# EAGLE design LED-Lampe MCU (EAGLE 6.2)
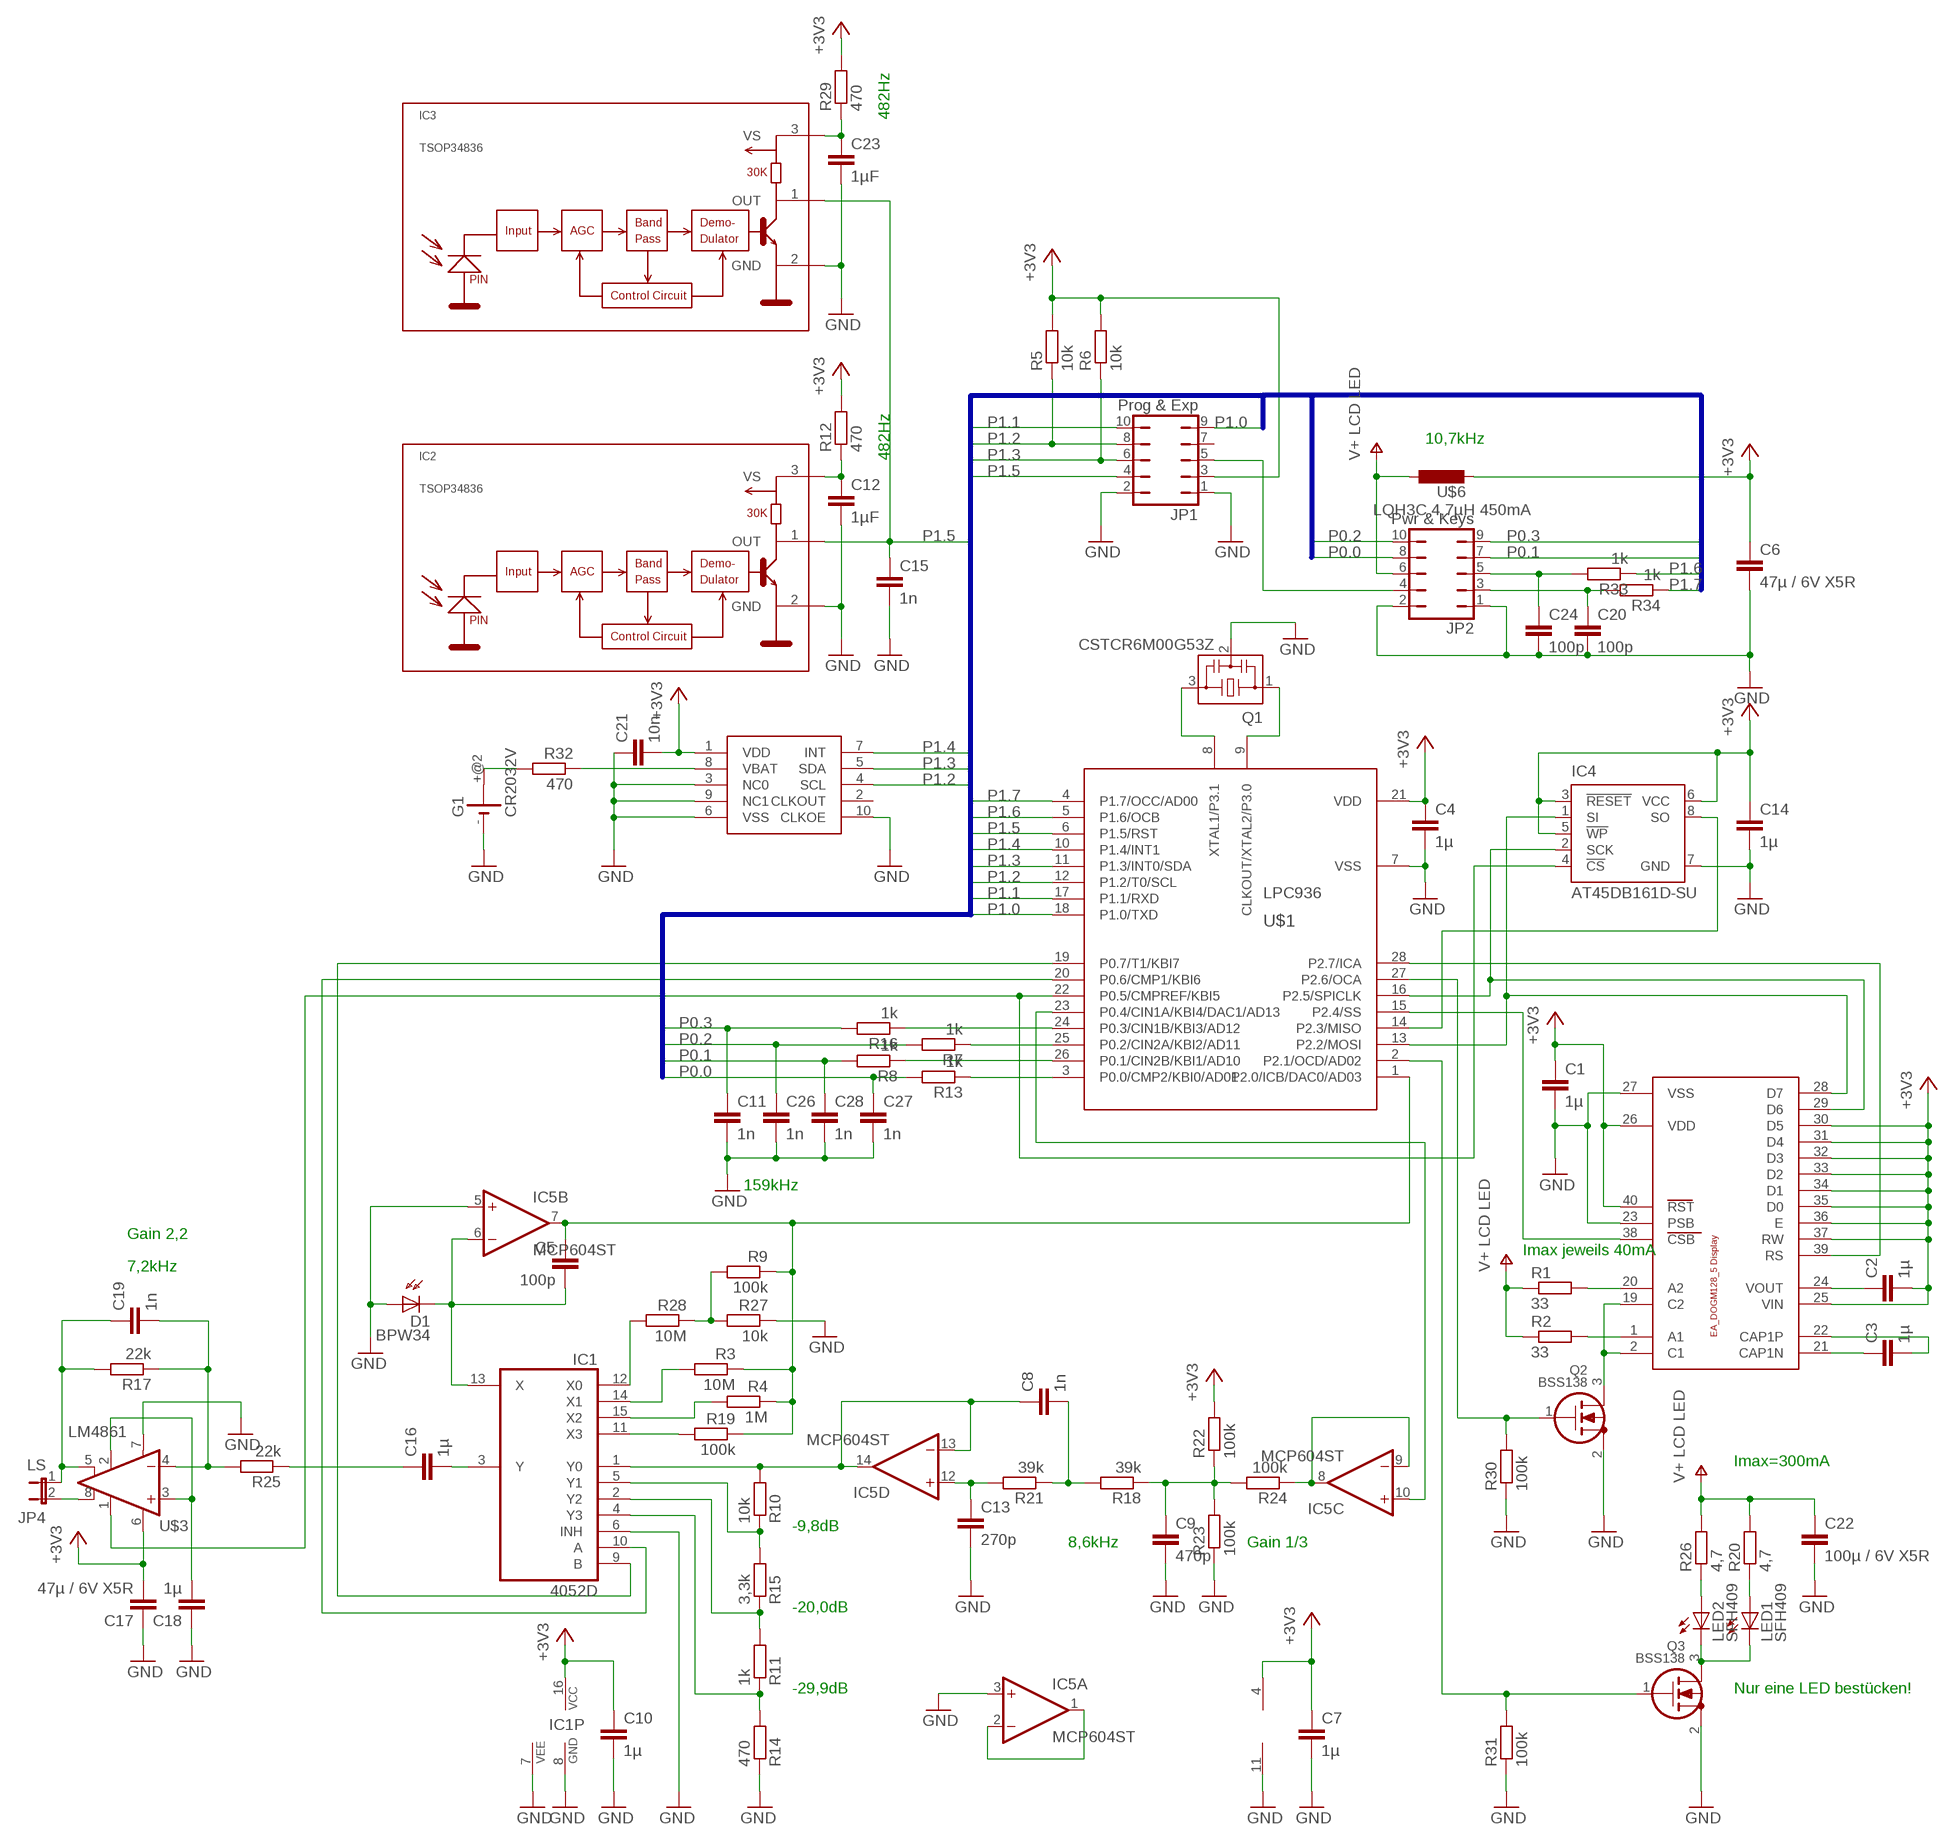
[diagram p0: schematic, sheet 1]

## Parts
C1  1µ  C-EUC0805  [C0805]
C2  1µ  C-EUC0805  [C0805]
C3  1µ  C-EUC0805  [C0805]
C4  1µ  C-EUC0805  [C0805]
C5  100p  C-EUC0603  [C0603]
C6  47µ / 6V X5R  C-EUC1206  [C1206]
C7  1µ  C-EUC0805  [C0805]
C8  1n  C-EUC0805  [C0805]
C9  470p  C-EUC0805  [C0805]
C10  1µ  C-EUC0805  [C0805]
C11  1n  C-EUC0603  [C0603]
C12  1µF  C-EUC0805  [C0805]
C13  270p  C-EUC0805  [C0805]
C14  1µ  C-EUC0805  [C0805]
C15  1n  C-EUC0603  [C0603]
C16  1µ  C-EUC1206  [C1206]
C17  47µ / 6V X5R  C-EUC1206  [C1206]
C18  1µ  C-EUC1206  [C1206]
C19  1n  C-EUC0805  [C0805]
C20  100p  C-EUC0603  [C0603]
C21  10n  C-EUC0805  [C0805]
C22  100µ / 6V X5R  C-EUC1206  [C1206]
C23  1µF  C-EUC0805  [C0805]
C24  100p  C-EUC0603  [C0603]
C26  1n  C-EUC0603  [C0603]
C27  1n  C-EUC0603  [C0603]
C28  1n  C-EUC0603  [C0603]
D1  BPW34  BPW32  [BPW32]
G1  CR2032V  [CR2032V]
IC1  4052D  [SO16]
IC2  TSOP34836  [TSOP348]
IC3  TSOP34836  [TSOP348]
IC4  AT45DB161D-SU  [8S2]
IC5  MCP604ST  [TSSOP14]
JP1  Prog & Exp  JP5Q  [JP5Q]
JP2  Pwr & Keys  JP5Q  [JP5Q]
JP4  LS  JP1E  [JP1]
LED1  SFH409  LED3MM  [LED3MM]
LED2  SFH409  LED3MM  [LED3MM]
Q1  CSTCR6M00G53Z  [CSTCR6M]
Q2  BSS138  [SOT23]
Q3  BSS138  [SOT23]
R1  33  R-EU_R1206  [R1206]
R2  33  R-EU_R1206  [R1206]
R3  10M  R-EU_R0805  [R0805]
R4  1M  R-EU_R0805  [R0805]
R5  10k  R-EU_R0805  [R0805]
R6  10k  R-EU_R0805  [R0805]
R7  1k  R-EU_R0805  [R0805]
R8  1k  R-EU_R0805  [R0805]
R9  100k  R-EU_R0805  [R0805]
R10  10k  R-EU_R0805  [R0805]
R11  1k  R-EU_R0805  [R0805]
R12  470  R-EU_R0805  [R0805]
R13  1k  R-EU_R0805  [R0805]
R14  470  R-EU_R0805  [R0805]
R15  3,3k  R-EU_R0805  [R0805]
R16  1k  R-EU_R0805  [R0805]
R17  22k  R-EU_R0805  [R0805]
R18  39k  R-EU_R0805  [R0805]
R19  100k  R-EU_R0805  [R0805]
R20  4,7  R-EU_R1206  [R1206]
R21  39k  R-EU_R0805  [R0805]
R22  100k  R-EU_R0805  [R0805]
R23  100k  R-EU_R0805  [R0805]
R24  100k  R-EU_R0805  [R0805]
R25  22k  R-EU_R0805  [R0805]
R26  4,7  R-EU_R1206  [R1206]
R27  10k  R-EU_R0805  [R0805]
R28  10M  R-EU_R0805  [R0805]
R29  470  R-EU_R0805  [R0805]
R30  100k  R-EU_R0805  [R0805]
R31  100k  R-EU_R0805  [R0805]
R32  470  R-EU_R0805  [R0805]
R33  1k  R-EU_R0805  [R0805]
R34  1k  R-EU_R0805  [R0805]
U$1  LPC936  [TSSOP28]
U$2  EA_DOGM162  [E_DOG-M162]
U$3  LM4861  [SO08]
U$4  RV3029-C2  [MC_RTC]
U$6  LQH3C 4,7µH 450mA  LQH3C  [L1210]

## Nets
+3V3: C1.1 C2.2 C4.1 C6.1 C7.1 C10.1 C14.1 C17.2 C21.2 IC1.16(VCC) IC4.3(!RESET) IC4.5(!WP) IC4.6(VCC) IC5.4(P:V+) JP1.3 R5.2 R6.2 R12.2 R22.2 R29.2 U$1.21(VDD) U$2.25(VIN) U$2.26(VDD) U$2.30(D5) U$2.31(D4) U$2.32(D3) U$2.33(D2) U$2.34(D1) U$2.35(D0) U$2.36(E) U$2.37(RW) U$2.40(RST) U$3.6(VDD) U$4.1(VDD) U$6.2
GND: C1.2 C4.2 C6.2 C7.2 C9.2 C10.2 C11.2 C12.2 C13.2 C14.2 C15.2 C17.1 C18.1 C20.2 C21.1 C22.2 C23.2 C24.2 C26.2 C27.2 C28.2 D1.A G1.- IC1.6(INH) IC1.7(VEE) IC1.8(GND) IC2.2(GND) IC3.2(GND) IC4.7(GND) IC5.3(A:+IN) IC5.5(B:+IN) IC5.11(P:V-) JP1.1 JP1.2 JP2.1 JP2.2 Q1.2 Q2.2(S) Q3.2(S) R14.1 R23.1 R27.1 R30.1 R31.1 U$1.7(VSS) U$2.23(PSB) U$2.27(VSS) U$3.7(GND) U$4.3(NC0) U$4.6(VSS) U$4.9(NC1) U$4.10(CLKOE)
N$1: C2.1 U$2.24(VOUT)
N$2: IC1.9(B) U$1.19(P0.7/T1/KBI7)
N$3: C3.2 U$2.22(CAP1P)
N$4: C3.1 U$2.21(CAP1N)
N$5: U$1.15(P2.4/SS) U$2.38(CSB)
N$6: C12.1 IC2.3(VS) R12.1
N$7: R1.2 U$2.20(A2)
N$8: R2.2 U$2.1(A1)
N$9: IC4.2(SCK) U$1.16(P2.5/SPICLK) U$2.29(D6)
N$10: IC4.1(SI) U$1.13(P2.2/MOSI) U$2.28(D7)
N$11: Q2.1(G) R30.2 U$1.27(P2.6/OCA)
N$12: IC1.10(A) U$1.20(P0.6/CMP1/KBI6)
N$13: U$1.28(P2.7/ICA) U$2.39(RS)
N$14: Q1.3 U$1.8(XTAL1/P3.1)
N$15: Q1.1 U$1.9(CLKOUT/XTAL2/P3.0)
N$16: Q2.3(D) U$2.2(C1) U$2.19(C2)
N$17: R8.1 U$1.26(P0.1/CIN2B/KBI1/AD10)
N$18: JP4.2 U$3.8(VO2)
N$19: R16.1 U$1.24(P0.3/CIN1B/KBI3/AD12)
N$20: R13.1 U$1.3(P0.0/CMP2/KBI0/AD01)
N$21: C18.2 U$3.2(BYPASS) U$3.3(+IN)
N$22: R7.1 U$1.25(P0.2/CIN2A/KBI2/AD11)
N$23: IC4.8(SO) U$1.14(P2.3/MISO)
N$25: IC1.4(Y3) R11.1 R14.2
N$26: IC1.2(Y2) R11.2 R15.1
N$27: IC1.5(Y1) R10.1 R15.2
N$28: C8.1 IC1.1(Y0) IC5.13(D:-IN) IC5.14(D:OUT) R10.2
N$29: C13.1 IC5.12(D:+IN) R21.2
N$30: C8.2 R18.2 R21.1
N$31: LED2.A R26.1
N$32: IC5.10(C:+IN) U$1.23(P0.4/CIN1A/KBI4/DAC1/AD13)
N$33: C5.2 D1.K(C) IC1.13(X) IC5.6(B:-IN)
N$34: C5.1 IC5.7(B:OUT) R3.1 R4.1 R9.1 R19.1 U$1.1(P2.0/ICB/DAC0/AD03)
N$35: IC1.11(X3) R19.2
N$36: C9.1 R18.1 R22.1 R23.2 R24.2
N$37: Q3.1(G) R31.2 U$1.2(P2.1/OCD/AD02)
N$38: IC1.15(X2) R4.2
N$39: IC1.14(X1) R3.2
N$40: IC1.12(X0) R28.2
N$41: C19.2 R17.1 R25.2 U$3.4(-IN)
N$42: C16.1 R25.1
N$43: JP1.5 JP2.4
N$44: C16.2 IC1.3(Y)
N$45: C19.1 JP4.1 R17.2 U$3.5(VO1)
N$46: LED1.K(C) LED2.K(C) Q3.3(D)
N$47: IC4.4(!CS) U$1.22(P0.5/CMPREF/KBI5) U$3.1(SHUTDOWN)
N$48: LED1.A R20.1
N$49: R32.1 U$4.8(VBAT)
N$50: R9.2 R27.2 R28.1
N$51: IC5.8(C:OUT) IC5.9(C:-IN) R24.1
N$52: G1.+@2(+) R32.2
N$53: IC5.1(A:OUT) IC5.2(A:-IN)
N$54: C23.1 IC3.3(VS) R29.1
N$55: C24.1 JP2.5 R33.2
N$56: C20.1 JP2.3 R34.2
P0.0: C27.1 JP2.8 R13.2
P0.1: C28.1 JP2.7 R8.2
P0.2: C26.1 JP2.10 R7.2
P0.3: C11.1 JP2.9 R16.2
P1.0: JP1.9 U$1.18(P1.0/TXD)
P1.1: JP1.10 U$1.17(P1.1/RXD)
P1.2: JP1.8 R5.1 U$1.12(P1.2/T0/SCL) U$4.4(SCL)
P1.3: JP1.6 R6.1 U$1.11(P1.3/INT0/SDA) U$4.5(SDA)
P1.4: U$1.10(P1.4/INT1) U$4.7(INT)
P1.5: C15.1 IC2.1(OUT) IC3.1(OUT) JP1.4 U$1.6(P1.5/RST)
P1.6: R33.1 U$1.5(P1.6/OCB)
P1.7: R34.1 U$1.4(P1.7/OCC/AD00)
V+: C22.1 JP2.6 R1.1 R2.1 R20.2 R26.2 U$6.1 ; supply symbol labelled V+ LCD LED
Unconnected: G1.+ JP1.7 U$4.2(CLKOUT)

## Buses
P1.[0..7],P0.[0..7]

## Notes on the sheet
- 482Hz
- 10,7kHz
- 482Hz
- 159kHz
- Gain 2,2
- Imax jeweils 40mA
- 7,2kHz
- Imax=300mA
- -9,8dB
- 8,6kHz | Gain 1/3
- -20,0dB
- -29,9dB | Nur eine LED bestücken!

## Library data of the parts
C1-C5 C7-C21 C23 C24 C26-C28 = rcl:C-EU: CAPACITOR, European symbol
C6 C22 = resistor:C-EU: CAPACITOR, European symbol
D1 = opto-trans-siemens:BPW32: PHOTO DIODE; OC_FARNELL: unknown; OC_NEWARK: unknown
G1 = battery:CR2032V: LI BATTERY Varta
IC1 = 40xx:4052: Dual 4-channel ANALOG MULTIPLEXER
IC2 IC3 = vishay-1:TSOP348*: IR Receiver Modules for Remote Control Systems http://www.vishay.com/ir-receiver-modules/
IC4 = atmel:AT45DB161D: 16-megabit 2.5V or 2.7V DataFlash Source: http://www.atmel.com/dyn/resources/prod_documents/doc3500.pdf; MF: ATMEL; MPN: AT45DB161D-SU; OC_FARNELL: 1455040
IC5 = linear:MCP604: Quad Op Amp 2.7V to 6.0V Single Supply CMOS Source: http://ww1.microchip.com/downloads/en/DeviceDoc/21314g.pdf
JP1 JP2 = jumper:JP5Q: JUMPER
JP4 = jumper:JP1E: JUMPER
LED1 LED2 = led:LED: LED
Q1 = murata-filter:CSTCR: Resonator Source: murata.co.jp; MPN: CSTCR6M00G53-R0; OC_FARNELL: 1170434; OC_NEWARK: 25M8759
Q2 Q3 = transistors:BSS138: BSS138: N-channel enhancement MOSFET (ON Semiconductor) 50V Uds, 200mA Id, 225mW Ptot, 3.5&Omega; Rdson
R1 R2 R5-R8 R12 R13 R16-R18 R20-R26 R29-R31 R33 R34 = rcl:R-EU_: RESISTOR, European symbol
R3 R4 R9-R11 R14 R15 R19 R27 R28 R32 = resistor:R-EU_: RESISTOR, European symbol
U$1 = nxp:LPC936
U$2 = display_ea_dog:EA_DOGM162
U$3 = LM4861:LM4861
U$4 = MicroCrystal:RV3029-C2
U$6 = mcl:LQH3C: muRata Chip Coil

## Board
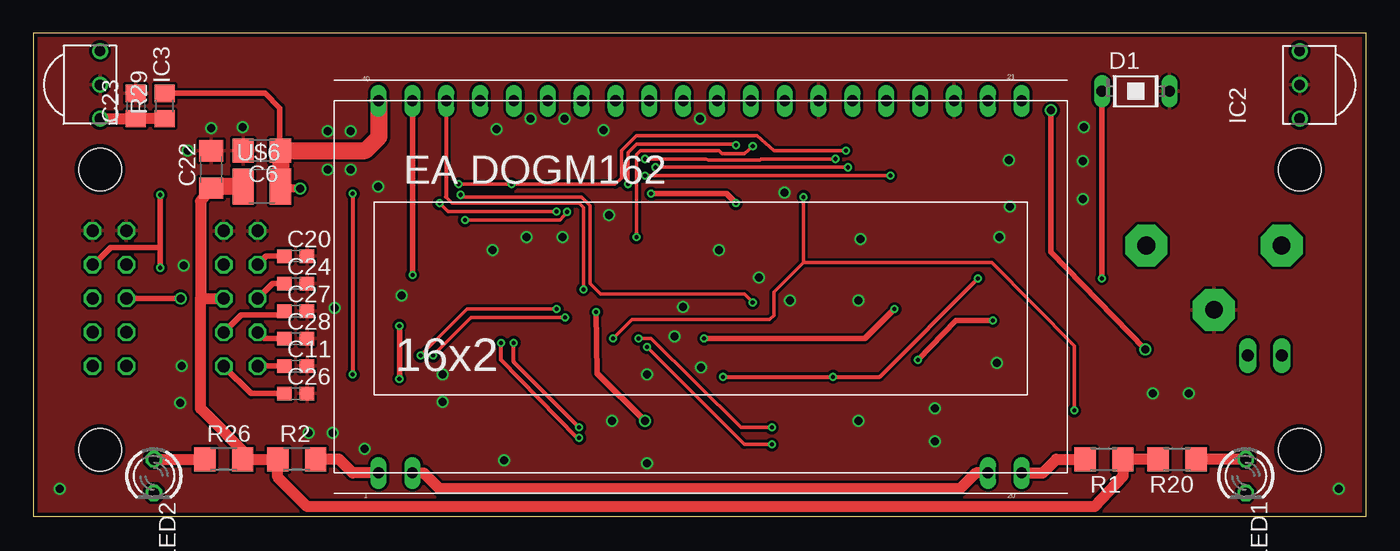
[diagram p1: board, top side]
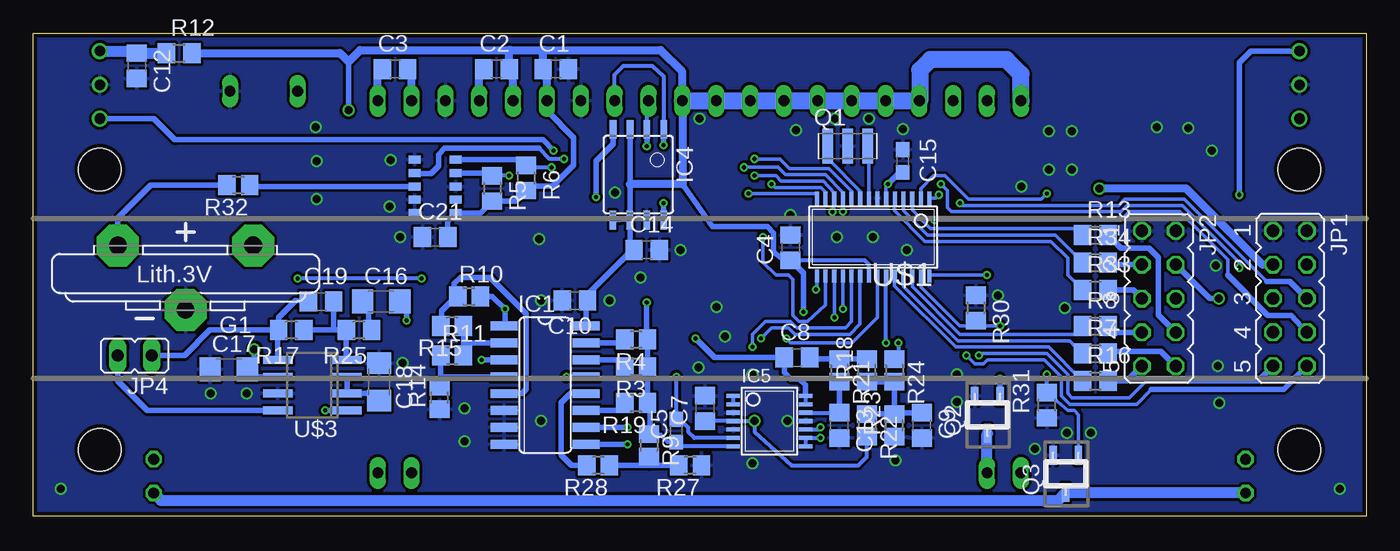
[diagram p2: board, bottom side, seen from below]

Size 100 x 36.25 mm. Coordinates in mm from the lower left corner, seen from the top.
Outline: 0,0 100,0 100,36.26 0,36.26 0,0
Copper layers (1*16): Top 0.035mm / dielectric 1.5mm / Bottom 0.035mm
Design rules: minimum track width 0.15mm, minimum drill 0.3mm, track to track 0.15mm, track to pad 0.15mm, pad to pad 0.15mm, via to via 0.15mm, smd to smd 0.15mm, copper to edge 0.3mm, drill to drill 0.2mm, minimum pad ring 0.2mm, minimum via ring 0.15mm, stop-mask expansion 0.075mm, vias tented up to drill 0mil, thermal gap 0.2mm
Holes 3.2 mm at 5,5 5,26.04 95,26.04 95,5

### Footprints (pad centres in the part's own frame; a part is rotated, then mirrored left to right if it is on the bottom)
C0805 = smd 1.3 x 1.5: 1 -0.95,0; 2 0.95,0
C0603 = smd 1.1 x 1: 1 -0.85,0; 2 0.85,0
C1206 = smd 1.6 x 1.8: 1 -1.4,0; 2 1.4,0
BPW32 = drill 0.813 long: A 0,2.54; K 0,-2.54
CR2032V = drill 1.321 pad 3.15 octagon: + -2.54,5.08; +@2 -2.54,-5.08; - 2.286,0
SO16 = smd 0.66 x 2.032: 1 -4.445,-3.073; 2 -3.175,-3.073; 3 -1.905,-3.073; 4 -0.635,-3.073; 5 0.635,-3.073; 6 1.905,-3.073; 7 3.175,-3.073; 8 4.445,-3.073; 9 4.445,3.073; 10 3.175,3.073; 11 1.905,3.073; 12 0.635,3.073; 13 -0.635,3.073; 14 -1.905,3.073; 15 -3.175,3.073; 16 -4.445,3.073
TSOP348 = drill 0.8: 1 -2.54,0; 2 0,0; 3 2.54,0
8S2 = smd 0.5 x 1.4: 1 -1.905,-3.404; 2 -0.645,-3.404; 3 0.625,-3.404; 4 1.895,-3.404; 5 1.905,3.404; 6 0.635,3.404; 7 -0.635,3.404; 8 -1.905,3.404
TSSOP14 = smd 0.305 x 0.991: 1 -1.905,-2.718; 2 -1.27,-2.718; 3 -0.635,-2.718; 4 0,-2.718; 5 0.635,-2.718; 6 1.27,-2.718; 7 1.905,-2.718; 8 1.905,2.718; 9 1.27,2.718; 10 0.635,2.718; 11 0,2.718; 12 -0.635,2.718; 13 -1.27,2.718; 14 -1.905,2.718
JP5Q = drill 0.914 octagon: 1 -5.08,-1.27; 2 -5.08,1.27; 3 -2.54,-1.27; 4 -2.54,1.27; 5 0,-1.27; 6 0,1.27; 7 2.54,-1.27; 8 2.54,1.27; 9 5.08,-1.27; 10 5.08,1.27
JP1 = drill 0.914 long: 1 0,-1.27; 2 0,1.27
LED3MM = drill 0.813 octagon: A -1.27,0; K 1.27,0
CSTCR6M = smd 0.8 x 2.6: 1 -1.5,0; 2 0,0; 3 1.5,0
SOT23 = smd 0.55 x 1.4: 1 0.95,1.4; 2 -0.95,1.4; 3 0,-1.4
R1206 = smd 1.6 x 1.803: 1 -1.422,0; 2 1.422,0
R0805 = smd 1.3 x 1.5: 1 -0.85,0; 2 0.85,0
R0805' = smd 1.3 x 1.5: 1 -0.95,0; 2 0.95,0
TSSOP28 = smd 0.305 x 0.991: 1 -4.225,-2.918; 2 -3.575,-2.918; 3 -2.925,-2.918; 4 -2.275,-2.918; 5 -1.625,-2.918; 6 -0.975,-2.918; 7 -0.325,-2.918; 8 0.325,-2.918; 9 0.975,-2.918; 10 1.625,-2.918; 11 2.275,-2.918; 12 2.925,-2.918; 13 3.575,-2.918; 14 4.225,-2.918; 15 4.225,2.918; 16 3.575,2.918; 17 2.925,2.918; 18 2.275,2.918; 19 1.625,2.918; 20 0.975,2.918; 21 0.325,2.918; 22 -0.325,2.918; 23 -0.975,2.918; 24 -1.625,2.918; 25 -2.275,2.918; 26 -2.925,2.918; 27 -3.575,2.918; 28 -4.225,2.918
E_DOG-M162 = drill 0.8 long: 1 -24.098,-13.97; 2 -21.558,-13.97; 19 21.622,-13.97; 20 24.162,-13.97; 21 24.162,13.97; 22 21.622,13.97; 23 19.082,13.97; 24 16.542,13.97; 25 14.002,13.97; 26 11.462,13.97; 27 8.922,13.97; 28 6.382,13.97; 29 3.842,13.97; 30 1.302,13.97; 31 -1.238,13.97; 32 -3.778,13.97; 33 -6.318,13.97; 34 -8.858,13.97; 35 -11.398,13.97; 36 -13.938,13.97; 37 -16.478,13.97; 38 -19.018,13.97; 39 -21.558,13.97; 40 -24.098,13.97
SO08 = smd 0.6 x 2.2: 1 -1.905,-2.6; 2 -0.635,-2.6; 3 0.635,-2.6; 4 1.905,-2.6; 5 1.905,2.6; 6 0.635,2.6; 7 -0.635,2.6; 8 -1.905,2.6
MC_RTC = smd 0.6 x 0.899: 1 -2,-1.549; 2 -1,-1.549; 3 0,-1.549; 4 1,-1.549; 5 2,-1.549; 6 2,1.549; 7 1,1.549; 8 0,1.549; 9 -1,1.549; 10 -2,1.549
L1210 = smd 1.6 x 2.7: 1 -1.4,0; 2 1.4,0

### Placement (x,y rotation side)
C1  60.8,33.58 0 bottom
C2  65.25,33.58 0 bottom
C3  72.87,33.58 0 bottom
C4  43.18,20.16 90 bottom
C5  51.75,6.43 90 bottom
C6  17.14,27.46 180 top
C7  49.61,8.1 90 bottom
C8  42.7,11.91 0 bottom
C9  33.34,6.83 270 bottom
C10  59.37,16.19 180 bottom
C11  19.68,11.27 0 top
C12  92.23,33.81 270 bottom
C13  39.53,6.83 270 bottom
C14  53.98,20 0 bottom
C15  34.77,26.67 90 bottom
C16  73.9,16.11 0 bottom
C17  85.33,11.03 0 bottom
C18  74.06,10.08 270 bottom
C19  78.42,16.11 0 bottom
C20  19.68,19.53 0 top
C21  69.85,20.95 0 bottom
C22  13.34,26.04 90 top
C23  7.7,30.8 90 top
C24  19.68,17.46 0 top
C26  19.68,9.21 0 top
C27  19.68,15.4 0 top
C28  19.68,13.34 0 top
D1  82.71,31.91 270 top
G1  88.58,17.78 270 bottom
IC1  61.59,9.84 270 bottom
IC2  95,32.38 90 top
IC3  5,32.38 270 top
IC4  54.61,25.64 180 bottom
IC5  44.77,7.14 270 bottom
JP1  5.71,16.36 270 bottom
JP2  15.56,16.35 270 bottom
JP4  92.39,12.06 90 bottom
LED1  90.96,3.02 270 top
LED2  9.05,3.02 270 top
Q1  38.89,27.78 0 bottom
Q2  28.42,7.62 0 bottom
Q3  22.54,3.17 0 bottom
R1  80.33,4.29 180 top
R2  19.76,4.29 0 top
R3  54.77,11.19 180 bottom
R4  54.77,13.26 180 bottom
R5  10k  [R0805']  65.56,24.61 270 bottom
R6  10k  [R0805']  63.02,25.4 270 bottom
R7  1k  [R0805']  20.32,12.22 0 bottom
R8  1k  [R0805']  20.32,14.29 0 bottom
R9  53.82,5.32 270 bottom
R10  67.31,16.51 0 bottom
R11  68.58,12.06 0 bottom
R12  470  [R0805']  89.06,34.77 0 bottom
R13  1k  [R0805']  20.32,21.11 0 bottom
R14  69.53,8.89 90 bottom
R15  68.58,14.29 180 bottom
R16  1k  [R0805']  20.32,10.16 0 bottom
R17  22k  [R0805']  80.64,13.97 180 bottom
R18  37.47,10.95 90 bottom
R19  54.77,8.49 180 bottom
R20  85.8,4.29 180 top
R21  39.53,10.95 270 bottom
R22  37.47,6.83 270 bottom
R23  35.4,6.83 90 bottom
R24  35.4,10.95 270 bottom
R25  22k  [R0805']  75.56,13.97 180 bottom
R26  14.29,4.29 0 top
R27  50.72,3.81 180 bottom
R28  57.63,3.81 180 bottom
R29  470  [R0805']  9.84,30.8 90 top
R30  100k  [R0805']  29.29,15.64 270 bottom
R31  100k  [R0805']  23.97,8.33 90 bottom
R32  84.61,24.84 180 bottom
R33  1k  [R0805']  20.32,16.99 0 bottom
R34  1k  [R0805']  20.32,19.05 0 bottom
U$1  36.99,20.95 180 bottom
U$2  50,17.23 0 top
U$3  79.06,9.84 90 bottom
U$4  69.85,24.77 90 bottom
U$6  17.14,24.77 0 top

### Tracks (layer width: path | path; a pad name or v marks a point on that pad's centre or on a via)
+3V3  (via drill 0.3, 0.6)
  Top 0.406: 18.57,25.21 U$6.2 | v45.88,7.14 42.31,10.72 v42.23,15.33 | v83.42,12.54 76.36,19.84 v76.36,30.48 | R29.2 17.39,31.75 18.49,30.64 18.49,27.51 C6.1
  Top 0.61: v20,24.61 19.05,24.61 18.57,25.21
  Top 1.27: U$6.2 C6.1 24.92,27.46 25.93,28.47 25.93,31.04 U$2.40
  Bottom 0.152: 51.28,31.91 51.28,32.07 U$2.30 | 55.33,22.31 IC4.6 | 33.5,31.2 U$2.37 | 42.7,18.73 C4.1 | 55.24,20.16 54.92,20.16 C14.1
  Bottom 0.305: U$1.21 37.31,18.9 37.62,19.21 C4.1 | 76.36,34.13 | R22.2 37.47,4.45 38.1,3.81 43.1,3.81 45.88,6.35 v45.88,7.14 IC5.4 49.45,7.14 C7.1
  Bottom 0.406: IC4.5 55.33,22.31 IC4.6 | C14.1 55.24,20.16 IC4.6 55.24,24.92 55.24,29.11 IC4.3 | C17.2 83.66,10.48 U$3.6 83.66,10.48 83.42,10.56 v83.42,12.54 | IC1.16 58.52,16.09 C10.1 58.42,16.67 55.24,19.84 55.24,20.16 | R5.2 66.45,22.77 U$4.1 68.9,22.17 C21.2 | C4.1 43.66,19.21 44.45,19.84 44.45,21.27 44.93,21.75 49.05,21.75 51.28,24.92 | v42.23,15.33 42.23,18.26 42.7,18.73 | v76.36,30.48 76.36,34.13 | R5.2 | R5.2 63.82,23.65 R6.2 62.71,24.77 61.04,24.77 59.45,26.35 59.45,28.42 61.44,30.4 61.44,31.17 U$2.26
  Bottom 0.61: U$2.30 51.3,33.36 52.94,35 61.67,35 | 51.28,31.91 51.28,24.92 55.24,24.92 | 64.21,35 75.49,35 76.36,34.13 76.99,34.77 R12.2 | 64.21,35 61.67,35 | v20,24.61 13.49,24.61 7.78,18.89 JP1.3 | 64.21,35 64.3,35.01 C2.2 64,33.36 U$2.25 | U$2.26 61.46,33.47 C1.1 61.75,35 61.67,35
  Bottom 1.27: U$2.30 U$2.31 U$2.32 U$2.33 U$2.34 U$2.35 U$2.36 U$2.37 | U$2.40 25.9,33.2 26.99,34.29 32.7,34.29 33.5,33.5 33.5,31.2 33.5,31.19
GND  (via drill 0.6)
  other vias: 15.72,29.21 78.82,29.21 22.07,28.89 13.34,29.13 54.45,17.94 56.75,16.19 36.99,20.95 43.18,22.62 25.88,24.77 27.62,16.59 22.07,26.04 11.59,27.46 35.32,4.21 11.11,11.27 11.03,8.49 30.72,10.64 24.84,5.08 30.72,8.57 46.04,10.64 50.09,11.19 48.74,15.72 48.1,13.49 61.91,16.19 72.47,20.95 51.44,20 86.68,9.21 83.98,9.21 61.91,7.14 72.31,11.51 23.81,26.04 1.98,2.06 73.18,26.75 73.26,23.26 39.69,20.95 34.45,20 34.77,29.05 42.78,28.97 39.85,29.84 37.31,29.84 56.36,24.29 50.01,29.84 62.07,20.8 46.04,3.97 11.27,18.81 20.64,6.27 22.46,6.27 22.62,15.64 67.63,5.64 67.63,8.1 97.95,2.06 78.74,23.81 78.74,26.67 23.81,28.89 43.42,7.14
  pour Top (isolate 0.203): 0,36.25 100,36.25 100,0 0,0
  pour Bottom (isolate 0.203): 0,0 100.01,0 100.01,36.25 0,36.25
N$1
  Bottom 0.61: U$2.24 66.54,33.07 C2.1
N$2  (via drill 0.3)
  Top 0.254: v55.4,5.4 53.34,5.4 v46.04,12.7
  Bottom 0.152: 38.6,18 U$1.19
  Bottom 0.254: v46.04,12.7 46.04,13.65 45.09,14.61 43.18,14.61 42.7,14.13 39.05,14.13 38.6,14.61 38.6,18
  Bottom 0.406: IC1.9 v55.4,5.4
N$3
  Bottom 0.61: U$2.22 71.62,33.36 C3.2
N$4
  Bottom 0.61: U$2.21 74.16,33.23 C3.1
N$5  (via drill 0.3)
  Top 0.152: U$2.38 31.01,31.33 30.96,31.27
  Top 0.254: 30.96,23.97 31.43,23.5 40.96,23.5 41.27,23.18 v41.27,17.04
  Top 0.305: 30.96,31.27 30.96,23.97
  Bottom 0.254: U$1.15 41.21,17.05 v41.27,17.04
N$6
  Bottom 0.813: IC2.3 92.32,34.92 C12.1 R12.1
N$7
  Top 0.813: U$2.20 75.73,3.26 76.76,4.29 R1.2
N$8
  Top 0.813: U$2.1 23.97,3.26 22.94,4.29 R2.2
N$9  (via drill 0.3 pad 0.3)
  Top 0.254: v53.98,27.78 53.34,27.23 51.67,27.23 51.44,27.46 45.56,27.46 45.24,27.15 v45.24,20.95
  Bottom 0.152: 53.97,27.79 v53.98,27.78 | 40.56,17.93 U$1.16
  Bottom 0.254: v45.24,20.95 45.24,19.05 44.29,18.1 43.34,18.1 43.02,17.78 43.02,15.08 42.55,14.61 41.91,14.61 40.56,15.85 40.56,17.93
  Bottom 0.305: IC4.2 53.97,31.1 U$2.29
  Bottom 0.406: IC4.2 53.97,27.79
N$10  (via drill 0.3 pad 0.3)
  Top 0.254: v44.61,24.92 44.61,27.3 45.24,27.94 52.63,27.94 v52.7,27.86
  Bottom 0.254: 52.7,29.21 IC4.1 | U$1.13 40.56,24.32 40.9,24.69 44.37,24.69 v44.61,24.92
  Bottom 0.305: U$2.28 56.38,33.15 55.72,33.81 53.58,33.81 52.7,33.02 52.7,29.21
  Bottom 0.406: v52.7,27.86 52.7,29.21
N$11  (via drill 0.3)
  Top 0.406: v27.46,10.32 v27.46,14.29
  Bottom 0.152: U$1.27 33.44,18.04
  Bottom 0.254: v27.46,14.29 29.37,14.29 30.48,14.29 33.41,17.22 33.41,18.02 33.44,18.04
  Bottom 0.305: R30.2 29.37,14.69 29.37,14.29
  Bottom 0.406: Q2.1 27.47,9.52 v27.46,10.32
N$12  (via drill 0.3)
  Top 0.254: v45.4,13.34 46.35,13.34 53.1,6.67 v55.4,6.67
  Bottom 0.152: U$1.20 37.96,18.07 37.97,18.1
  Bottom 0.254: v45.4,13.34 44.61,14.13 43.34,14.13 42.86,13.65 38.73,13.65 37.97,14.45 37.97,18.1
  Bottom 0.406: IC1.10 v55.4,6.67
N$13  (via drill 0.3)
  Top 0.406: v28.44,18.12 U$2.39
  Bottom 0.152: 32.68,18.12 U$1.28 | v28.44,18.12 28.42,18.1
  Bottom 0.254: 32.68,18.12 v28.44,18.12
N$14
  Bottom 0.152: 37.31,27.63 37.47,27.78 Q1.3
  Bottom 0.254: U$1.8 37.31,27.63
N$15
  Bottom 0.152: 40.32,26.78 40.32,27.71 Q1.1
  Bottom 0.254: U$1.9 37.96,24.42 40.32,26.78
N$16
  Top 0.813: U$2.19 70.73,3.26 69.53,2.06 30.48,2.06 29.29,3.26 U$2.2
  Bottom 0.813: U$2.2 28.44,6.2 Q2.3
N$17
  Bottom 0.152: R8.1 21.27,13.81 21.43,13.65 | 34.05,17.92 U$1.26
  Bottom 0.254: 21.43,13.65 30.48,13.65 34.05,17.25 34.05,17.92
N$18
  Bottom 0.406: JP4.2 93.66,10.16 91.44,7.94 U$3.8 81.6,7.94
N$19
  Bottom 0.152: R16.1 21.43,10.32 | U$1.24 35.36,18.06 35.38,18
  Bottom 0.254: 21.43,10.32 23.81,12.7 30.8,12.7 35.38,17.28 35.38,18
N$20
  Bottom 0.152: U$1.3 34.05,23.84
  Bottom 0.254: 34.05,23.84 34.05,22.99 32.7,21.59 21.75,21.59 R13.1
N$21
  Bottom 0.406: U$3.3 U$3.2 73.98,9.21 C18.2
N$22
  Bottom 0.152: R7.1 21.35,12.22 | 34.72,17.96 U$1.25
  Bottom 0.254: 21.35,12.22 22.23,13.18 30.64,13.18 34.72,17.25 34.72,17.96
N$23  (via drill 0.3, 0.3 pad 0.3)
  Top 0.406: v46.35,24.21 51.99,24.21 v52.7,23.5
  Bottom 0.152: U$1.14 41.21,24.07
  Bottom 0.254: 41.21,24.07 41.35,24.21 v46.35,24.21
  Bottom 0.406: v52.7,23.5 IC4.8
N$25
  Bottom 0.406: R11.1 69.43,10.32 | 69.43,10.32 69.43,9.84 R14.2 | IC1.4 69.27,10.48 69.43,10.32
N$26
  Bottom 0.406: IC1.2 67.63,13.02 67.63,12.17 R11.2 R15.1
N$27
  Bottom 0.406: IC1.5 63.34,9.21 63.02,9.53 63.02,15.24 65.72,17.94 67.94,17.94 68.42,17.46 68.42,16.57 R10.1 68.26,16.51 69.37,15.4 69.37,14.45 69.53,14.29 R15.2 69.37,14.29
N$28  (via drill 0.3)
  Top 0.406: v50.32,13.34 62.39,13.34 v64.61,15.56
  Bottom 0.305: IC5.13 IC5.14
  Bottom 0.406: R10.2 65.56,16.51 v64.61,15.56 | v64.61,15.56 64.61,14.35 IC1.1 | v50.32,13.34 48.9,11.91 C8.1 43.65,10.79 43.18,10.32 42.55,10.32 42.07,9.84 42.07,9.07 IC5.14 | v64.61,15.56 64.61,14.29
N$29
  Bottom 0.305: IC5.12 39.69,7.78 C13.1
  Bottom 0.406: 39.85,7.94 C13.1 R21.2
N$30
  Bottom 0.152: 42.07,11.91 41.91,11.91 41.75,11.8
  Bottom 0.254: 41.75,11.8 41.97,11.96
  Bottom 0.406: R18.2 R21.1 41.75,11.8 | C8.2 42.07,11.91
N$31
  Top 0.305: 12.78,4.29 R26.1
  Top 0.813: LED2.A 12.78,4.29
N$32  (via drill 0.3)
  Top 0.305: v40.96,6.67 36.04,11.59 v36.04,13.02
  Bottom 0.305: IC5.10 41.12,6.51 v40.96,6.67 | v36.04,13.02 36.04,18.1 U$1.23
N$33  (via drill 0.3)
  Top 0.305: v51.75,10.48 v60.01,10.48 63.5,10.48 v70.88,17.86
  Top 0.406: v80.17,17.86 D1.K
  Bottom 0.305: v70.88,17.86 v80.17,17.86 | v51.75,10.48 C5.2 51.49,7.28 50.88,6.67 50.88,6.35 50.4,5.87 IC5.6
  Bottom 0.406: v60.01,10.48 IC1.13
N$34  (via drill 0.3 pad 0.3)
  Top 0.254: v32.07,24.13 32.23,23.97 41.12,23.97 41.75,23.34 41.75,17.46 42.55,16.67 53.34,16.67 v53.98,16.03
  Bottom 0.152: 53.98,13.71 R4.1
  Bottom 0.254: U$1.1 32.27,23.87 v32.07,24.13
  Bottom 0.305: IC5.7 51.41,5.24 C5.1 52.41,5.58 52.94,6.11 53.76,6.11 R9.1
  Bottom 0.406: R4.1 R3.1 R19.1 53.74,8.49 53.74,6.19 R9.1 | v53.98,16.03 53.98,13.71
N$35
  Bottom 0.406: R19.2 56.12,7.94 IC1.11
N$36
  Bottom 0.406: 35.72,10.16 R24.2 | R18.1 R24.2 | R24.2 R23.2 | R23.2 R22.1 | C9.1 35.32,7.78 35.4,7.78 R23.2
N$37  (via drill 0.3)
  Top 0.305: v23.97,24.21 v23.97,10.64
  Bottom 0.254: U$1.2 33.41,24.61 32.46,25.56 31.59,25.56 29.84,23.81 24.37,23.81 v23.97,24.21 | R31.2 22.38,7.94 21.91,7.94 21.59,7.62 21.59,4.6
  Bottom 0.305: 21.59,4.6 Q3.1 | R31.2 v23.97,10.64
  Bottom 0.406: R31.2
N$38
  Bottom 0.406: IC1.15 55.8,13.02 R4.2
N$39
  Bottom 0.406: R3.2 55.88,11.59 55.88,11.75 IC1.14
N$40
  Bottom 0.406: R28.2 59.61,3.81 60.4,4.6 60.4,8.49 59.69,9.21 IC1.12
N$41
  Bottom 0.406: R17.1 R25.2 | C19.2 77.47,13.97 R25.2 | R25.2 76.52,11.8 U$3.4
N$42
  Bottom 0.406: R25.1 74.85,13.97 74.85,16.11 C16.1
N$43  (via drill 0.6)
  Top 0.406: JP1.5 v11.04,16.36
  Bottom 0.406: v11.04,16.36 11.75,16.35 JP2.4
N$44  (via drill 0.3)
  Top 0.406: v66.36,11.75 69.22,14.68 v71.99,14.68
  Bottom 0.406: IC1.3 v66.36,11.75 | v71.99,14.68 71.99,16.11 C16.2
N$45
  Bottom 0.406: U$3.5 81.66,13.91 R17.2 | R17.2 81.59,14.93 80.33,16.19 C19.1 | JP4.1 88.66,12.06 86.76,13.97 R17.2
N$46
  Bottom 0.813: LED2.K 22.51,1.75 Q3.3 22.57,1.75 23.1,1.19 90.41,1.19 LED1.K
N$47  (via drill 0.3)
  Top 0.254: v43.5,13.34 44.93,14.76 55.24,14.76 55.56,15.08 55.56,16.83 57.78,19.05 | 57.78,19.05 v57.78,23.97 | 57.78,19.05 71.91,19.05 78.11,12.78 v78.11,7.94
  Bottom 0.152: U$1.22 | IC4.4 56.51,29.06 IC4.4
  Bottom 0.254: U$1.22 36.66,14.93 38.58,13.02 43.18,13.02 v43.5,13.34
  Bottom 0.406: v57.78,23.97 57.78,26.67 56.52,27.94 IC4.4 | v78.11,7.94 U$3.1
N$48
  Top 0.813: LED1.A R20.1
N$49
  Bottom 0.406: U$4.8 83.68,24.77 R32.1
N$50
  Bottom 0.406: R27.2 53.74,3.81 | 53.74,3.81 R28.1 | R9.2 53.74,4.45 53.74,3.81
N$51  (via drill 0.3)
  Top 0.305: v40.96,5.87 40.8,5.87 35.08,11.75 v35.08,13.02
  Bottom 0.305: IC5.8 IC5.9 v40.96,5.87 | v35.08,13.02 35.08,11.8 R24.1
N$52
  Bottom 0.406: R32.2 91.2,24.84 93.66,22.38 G1.+@2
N$53
  Bottom 0.305: IC5.2 IC5.1
N$54
  Top 0.813: C23.1 | IC3.3 C23.1 | R29.1 C23.1
N$55
  Top 0.406: C24.1 17.94,17.46 JP2.5
  Bottom 0.406: JP2.5 17.46,16.98 R33.2
N$56
  Top 0.406: C20.1 17.47,19.53 JP2.3
  Bottom 0.406: JP2.3 18.9,18.89 R34.2
P0.0
  Top 0.406: 18.89,15.4 C27.1 18.78,15.4 18.49,15.11 15.59,15.11 JP2.8
  Bottom 0.406: JP2.8 15.6,15.12 15.6,19.43 16.31,20.14 18.4,20.14 R13.2
P0.1
  Top 0.152: JP2.7
  Top 0.406: C28.1 17.3,13.34 JP2.7
  Bottom 0.152: R8.2 | JP2.7 16.84,13.79
  Bottom 0.406: R8.2 18.89,13.81 JP2.7
P0.2
  Top 0.406: C26.1 16.35,9.21 JP2.10
  Bottom 0.152: 18.73,12.38 R7.2
  Bottom 0.406: JP2.10 15.4,12.38 18.73,12.38
P0.3
  Top 0.152: JP2.9
  Top 0.406: C11.1 JP2.9
  Bottom 0.406: JP2.9 17.94,10.16 R16.2
P1.0  (via drill 0.3, 0.3 pad 0.3)
  Top 0.254: v39.26,15.56 32.54,15.56 v29.05,12.06
  Bottom 0.152: 39.26,17.98 U$1.18 | v29.05,12.06 28.89,12.22
  Bottom 0.254: v39.26,15.56 39.26,17.98 | 28.89,12.22 23.97,12.22 22.38,10.64 22.38,9.21 22.07,8.89 17.78,8.89 16.51,10.16
  Bottom 0.406: 16.51,10.16 8.1,10.16 JP1.9
P1.1  (via drill 0.3, 0.3 pad 0.3)
  Top 0.254: v30,12.06 32.86,14.92 v39.9,14.92
  Bottom 0.152: 39.9,17.95 U$1.17 | JP1.10
  Bottom 0.254: v39.9,14.92 39.9,17.95 | 16.11,9.53 17.22,8.41 22.23,8.41 22.86,9.05 22.86,10.48 24.13,11.75 28.42,11.75 28.73,11.43 29.37,11.43 v30,12.06
  Bottom 0.406: JP1.10 6.19,9.53 16.11,9.53
P1.2  (via drill 0.3)
  Top 0.254: v64.29,25.56 v45.88,25.56 | v40.03,22.85 39.53,22.23 v32.38,22.23
  Bottom 0.152: 39.92,23.91 U$1.12 | 66.09,25.77 65.77,25.77 R5.1
  Bottom 0.254: v45.88,25.56 44.29,25.56 43.89,25.16 40.72,25.16 39.92,24.32 39.92,23.91 39.92,22.96 v40.03,22.85 | v32.38,22.23 18.41,22.23 17.78,22.86 13.97,22.86 10.4,19.29 10.4,18.1
  Bottom 0.305: v64.29,25.56 R5.1
  Bottom 0.406: U$4.4 66.09,25.77 | JP1.8 5.64,15.08 7.38,15.08 10.4,18.1
P1.3  (via drill 0.3)
  Top 0.254: v61.12,26.19 v46.67,26.19 | v39.26,22.89 32.07,22.86 31.11,22.86 v30.48,23.5
  Bottom 0.152: 63.5,26.51 | 39.26,23.93 U$1.11 | 63.5,26.51 R6.1 63.5,26.67 63.6,26.77 | 63.5,26.51 63.18,26.19
  Bottom 0.254: v46.67,26.19 44.13,26.19 43.58,25.64 40.56,25.64 39.26,24.32 39.26,23.93 v39.26,22.89 | v30.48,23.5 30.32,23.34 18.57,23.34 18.1,23.81 13.65,23.81 7.46,17.62
  Bottom 0.305: 63.18,26.19 v61.12,26.19
  Bottom 0.406: U$4.5 63.6,26.77 | JP1.6 5.71,17.62 7.46,17.62
P1.4  (via drill 0.3)
  Top 0.254: v45.88,26.83 50.48,26.83 50.64,26.75 54.53,26.75 54.61,26.83 v60.17,26.83
  Bottom 0.152: U$4.7 71.44,25.72
  Bottom 0.254: U$1.10 38.61,24.41 40.32,26.11 43.26,26.11 43.97,26.83 v45.88,26.83
  Bottom 0.305: v60.17,26.83 61.28,26.83 62.07,27.62
  Bottom 0.406: 62.07,27.62 69.14,27.62 69.61,27.15 69.61,26.27 70.17,25.72 71.44,25.72
P1.5  (via drill 0.3, 0.3 pad 0.3)
  Top 0.254: v60.96,27.46 55.56,27.46 54.29,28.57 45.24,28.57 44.13,27.46 44.13,25.4 43.66,24.92 v35.88,24.92 v31.91,24.92
  Top 0.406: v9.53,24.13 9.53,20.16 | JP1.4 4.52,18.89 5.79,20.16 9.53,20.16 | 9.53,20.16 v9.53,18.65
  Bottom 0.152: v35.88,24.92 36.01,24.88 | C15.1 34.92,25.88
  Bottom 0.254: v31.91,24.92 31.43,24.45 31.43,23.18 31.11,22.86 18.41,22.86 17.94,23.34 13.81,23.34 9.53,19.05 v9.53,18.65 | U$1.6 36.01,24.77 35.87,24.92 v35.87,24.92 v35.88,24.92
  Bottom 0.406: v60.96,27.46 61.75,28.26 89.38,28.26 90.96,29.84 IC2.1 | 34.92,25.88 v35.88,24.92 | IC3.1 8.65,34.92 9.53,34.05 v9.53,24.13
P1.6
  Bottom 0.152: U$1.5 35.36,23.85 35.38,23.81
  Bottom 0.254: 35.38,23.81 35.38,22.94 33.1,20.64 23.65,20.64 22.38,19.37 22.38,18.1 R33.1
P1.7
  Bottom 0.152: 34.72,23.85 U$1.4
  Bottom 0.254: 34.72,23.85 34.72,22.94 32.91,21.11 23.33,21.11 R34.1
V+
  Top 0.406: 13.46,24.77 C22.1
  Top 0.813: 12.54,16.35 JP2.6 | 12.54,16.35 12.54,8.1 16.35,4.29 | C22.1 12.54,23.65 12.54,16.35 | 16.35,4.29 R2.1 18.34,2.94 20.56,0.71 79.61,0.71 81.75,3.01 R1.1 R20.2 | R26.2 16.35,4.29
  Top 1.27: U$6.1 13.46,24.77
